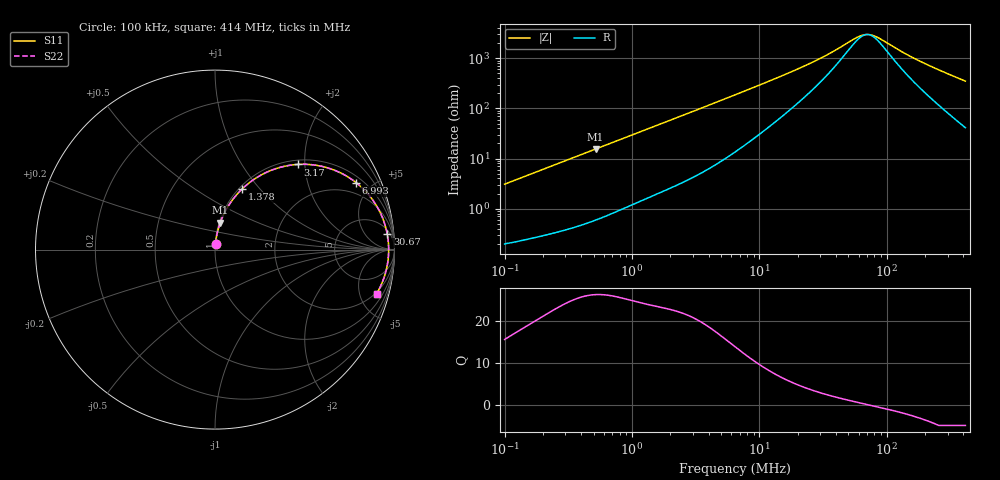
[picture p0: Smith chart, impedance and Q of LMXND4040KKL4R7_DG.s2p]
! LMXND4040KKL4R7_DG  S-PARAMETER MODEL  ( General Type )
! Model Generated by TAIYO YUDEN Corporation (http://www.ty-top.com)
! Version 1.0
! TAIYO YUDEN Control No. 191023NI43SB-FBB
! Copyright(c) 2019 TAIYO YUDEN CO.,LTD. All Rights Reserved.
! Product Description (link to TY-COMPAS)
! https://ds.yuden.co.jp/TYCOMPAS/or/detail?pn=LMXND4040KKL4R7MDG&u=M
! Products Name : Inductors
! Characteristics :
!  Inductance : 4.7 uH , SRF(min) : 47 MHz , DC Resistance(max) : 0.168 Ohm
!  Rated Current : Saturation :950 mA , Temp Rise : 1200 mA
!  Case Size : 4.0 x 4.0 / 0.157 x 0.157 [mm/inch] , Thickness : 1 / 0.039 [mm/inch]
!  (Conditions: Temperature = 25 degC , DC Bias Current/Voltage = 0A / 0V)
! External Node Assignments :
!  1  o---GGG---o  2
! GND o---------o GND
! Frequency Range : 0.1MHz  -  413.982163MHz  [ 402 STEP ]
# MHz S RI R 50
! Freq[MHz].  S11 Real  S11 Imag  S21 Real  S21 Imag  S12 Real  S12 Imag  S22 Real  S22 Imag
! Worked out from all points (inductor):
!   401 points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, 100 kHz to 414 MHz, reference 50 ohm
!   read as one part in series: L = 4.87 uH near 104.3 kHz
!   highest Q = 26.3 at 518 kHz (marker M1), where L = 4.77 uH
!   self-resonance near 70.25 MHz
!   S11 on the Smith chart (normalised r, x): 100 kHz: 1.00, +0.06; 1.378 MHz: 1.03, +0.81; 3.17 MHz: 1.09, +1.84; 6.993 MHz: 1.31, +4.05; 30.67 MHz: 8, +19; 414 MHz: 1.82, -6.97
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0.1  0.00291 0.0306  0.9971 -0.0306  0.9971 -0.0306  0.00291 0.0306
0.216058  0.00726 0.0649  0.9927 -0.0649  0.9927 -0.0649  0.00726 0.0649
0.403501  0.019 0.1184  0.981 -0.1184  0.981 -0.1184  0.019 0.1184
0.518029  0.029 0.1497  0.971 -0.1497  0.971 -0.1497  0.029 0.1497
0.890139  0.0736 0.242  0.9264 -0.242  0.9264 -0.242  0.0736 0.242
1.378317  0.1512 0.3379  0.8488 -0.3379  0.8488 -0.3379  0.1512 0.3379
1.628129  0.1954 0.3757  0.8046 -0.3757  0.8046 -0.3757  0.1954 0.3757
2.368389  0.3293 0.4478  0.6707 -0.4478  0.6707 -0.4478  0.3293 0.4478
3.169913  0.4601 0.4745  0.5399 -0.4745  0.5399 -0.4745  0.4601 0.4745
4.423099  0.6151 0.459  0.3849 -0.459  0.3849 -0.459  0.6151 0.459
6.434145  0.7613 0.3916  0.2387 -0.3916  0.2387 -0.3916  0.7613 0.3916
6.992953  0.7873 0.3724  0.2127 -0.3724  0.2127 -0.3724  0.7873 0.3724
12.26894  0.9029 0.2393  0.0971 -0.2393  0.0971 -0.2393  0.9029 0.2393
25.96183  0.9555 0.1068  0.0445 -0.1068  0.0445 -0.1068  0.9555 0.1068
30.66725  0.96 0.0851  0.04 -0.0851  0.04 -0.0851  0.96 0.0851
56.09266  0.9672 0.021  0.0328 -0.021  0.0328 -0.021  0.9672 0.021
66.25912  0.9677 0.00542  0.0323 -0.00542  0.0323 -0.00542  0.9677 0.00542
72.01376  0.9677 -0.00229  0.0323 0.00229  0.0323 0.00229  0.9677 -0.00229
79.9149  0.9676 -0.012  0.0324 0.012  0.0324 0.012  0.9676 -0.012
104.7562  0.9662 -0.0379  0.0338 0.0379  0.0338 0.0379  0.9662 -0.0379
191.6068  0.9555 -0.1079  0.0445 0.1079  0.0445 0.1079  0.9555 -0.1079
413.9822  0.9002 -0.2464  0.0998 0.2464  0.0998 0.2464  0.9002 -0.2464
